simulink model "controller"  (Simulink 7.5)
settings: Solver=FixedStepDiscrete  StartTime=0.0  StopTime=Inf  FixedStep=0.002  RelTol=1e-3
PostLoadFcn:
  | , if any(exist('dsrtsu_mdlpostloadfcn', 'file') == [2, 3, 6]), try dsrtsu_mdlpostloadfcn('Execute', bdroot); catch fprintf('Error in PostLoadFcn (dsrtsu_mdlpostloadfcn) for model "%s":
  |  %s
  | ', bdroot, lasterr); end, end,
libraries: rtilib1103 x5, simulink x1

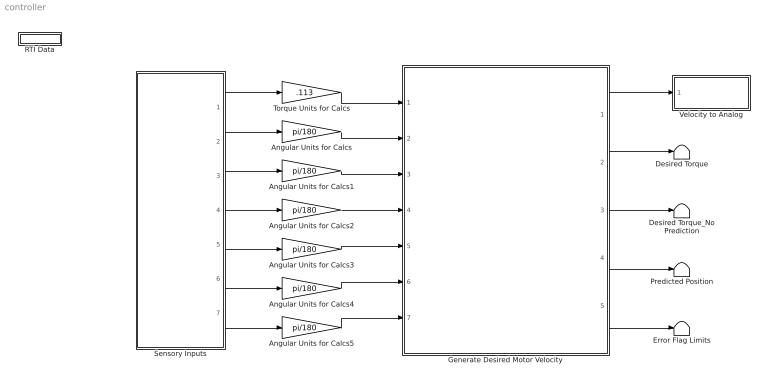
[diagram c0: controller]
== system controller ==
  Angular Units for Calcs{,1..5} (6 alike) : Gain  Gain=pi/180
  Desired Torque : Terminator
  Desired Torque_No Prediction : Terminator
  Error Flag Limits : Terminator
  Generate Desired Motor Velocity : Subsystem
  Predicted Position : Terminator
  RTI Data : Subsystem  Tag=struct('RTIDataServer',struct('RTIDataServerVs','2','RTIModelDescription','struct(''main'',''controller'',''sub'','''',''isMp'',0)'))  LoadFcn="if exist('rtidc'), try,  rtidc('DataHostBlockClbLoad', gcbh); catch, disp(['Warning: ''LoadFcn'' for RTI Data block failed: ' lasterr]); end, end,"
  Sensory Inputs : Subsystem
  Torque Units for Calcs : Gain  Gain=.113
  Velocity to Analog : Subsystem
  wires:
  Generate Desired Motor Velocity/1(Desired Velocity) -> Velocity to Analog/1(Velocity)
  Sensory Inputs/1(Ankle Torque) -> Torque Units for Calcs/1
  Sensory Inputs/2(Ankle Position) -> Angular Units for Calcs/1
  Sensory Inputs/3(Ankle Velocity) -> Angular Units for Calcs1/1
  Sensory Inputs/4(Sprocket Position) -> Angular Units for Calcs2/1
  Sensory Inputs/5(Sprocket Velocity) -> Angular Units for Calcs3/1
  Sensory Inputs/6(Motor Position) -> Angular Units for Calcs4/1
  Sensory Inputs/7(Motor Velocity) -> Angular Units for Calcs5/1
  Torque Units for Calcs/1 -> Generate Desired Motor Velocity/1(Ankle Torque)
  Angular Units for Calcs/1 -> Generate Desired Motor Velocity/2(Ankle Position)
  Angular Units for Calcs1/1 -> Generate Desired Motor Velocity/3(Ankle Velocity)
  Angular Units for Calcs2/1 -> Generate Desired Motor Velocity/4(Sprocket Position)
  Angular Units for Calcs3/1 -> Generate Desired Motor Velocity/5(Sprocket Velocity)
  Angular Units for Calcs4/1 -> Generate Desired Motor Velocity/6(Motor Position)
  Angular Units for Calcs5/1 -> Generate Desired Motor Velocity/7(Motor Velocity)
  Generate Desired Motor Velocity/2(Desired Torque) -> Desired Torque/1
  Generate Desired Motor Velocity/3(Desired Torque_No Prediction) -> Desired Torque_No Prediction/1
  Generate Desired Motor Velocity/4(Predicted Position) -> Predicted Position/1
  Generate Desired Motor Velocity/5(Error Flag_Limits) -> Error Flag Limits/1

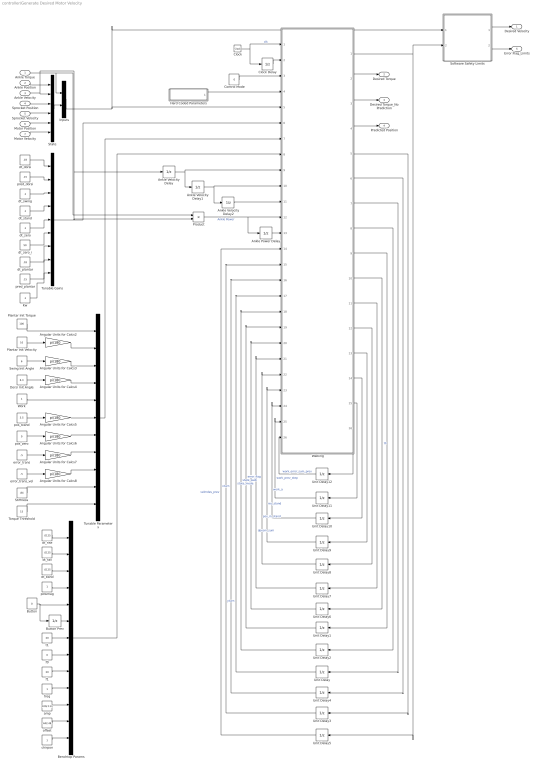
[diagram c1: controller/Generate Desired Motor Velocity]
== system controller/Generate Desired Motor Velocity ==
  Ankle Torque : Inport
  Ankle Position : Inport  Port=2
  Ankle Velocity : Inport  Port=3
  Sprocket Position : Inport  Port=4
  Sprocket Velocity : Inport  Port=5
  Motor Position : Inport  Port=6
  Motor Velocity : Inport  Port=7
  Angular Units for Calcs{2..8} (7 alike) : Gain  Gain=pi/180
  Ankle Power Delay : UnitDelay  SampleTime=0.002
  Ankle Velocity Delay : UnitDelay  SampleTime=0.002
  Ankle Velocity Delay1 : UnitDelay  SampleTime=0.002
  Ankle Velocity Delay2 : UnitDelay  SampleTime=0.002
  Benchtop Params : Mux  Inputs=13
  Button : Constant  Value=0
  Button Prev : UnitDelay  X0=1  SampleTime=0.002
  Clock : Clock
  Clock Delay : UnitDelay  SampleTime=0.002
  Control Mode : Constant  Value=0  SampleTime=.002
  Dorsi Init Angle : Constant  Value=6.3  SampleTime=.002
  Hard Coded Parameters : Stateflow chart  TreatAsAtomicUnit=on
  Inputs : Mux  Inputs=2
  Kw : Constant  Value=.1  SampleTime=.002
  Plantar Init Torque : Constant  Value=100  SampleTime=.002
  Plantar Init Velocity : Constant  Value=10  SampleTime=.002
  Product : Product  OutDataType=fixdt(1, 16)  OutScaling=2^0
  Software Safety Limits : Stateflow chart  TreatAsAtomicUnit=on
  State : Mux  Inputs=6
  Stiffness : Constant  Value=.84  SampleTime=.002
  Swing Init Angle : Constant  Value=6  SampleTime=.002
  Torque Threshold : Constant  Value=15  SampleTime=.002
  Tunable Gains : Mux  Inputs=9
  Tunable Parameters : Mux  Inputs=11
  Unit Delay{,1..12} (13 alike) : UnitDelay  SampleTime=0.002
  Walking : Stateflow chart  TreatAsAtomicUnit=on
  Work : Constant  SampleTime=.002
  amp : Constant  Value=100/.113  SampleTime=.002
  chirpon : Constant  SampleTime=.002
  dt_band : Constant  Value=.0125  SampleTime=.002
  dt_dorsi : Constant  Value=.03  SampleTime=.002
  dt_fall : Constant  Value=.0125  SampleTime=.002
  dt_plantar : Constant  Value=.03  SampleTime=.002
  dt_rise : Constant  Value=.0125  SampleTime=.002
  dt_stand : Constant  Value=.1  SampleTime=.002
  dt_swing : Constant  Value=.1  SampleTime=.002
  dt_zero : Constant  Value=.1  SampleTime=.002
  dt_zero_i : Constant  Value=50  SampleTime=.002
  error_trans : Constant  Value=.5  SampleTime=.002
  error_trans_vel : Constant  Value=.5  SampleTime=.002
  f0 : Constant  Value=0  SampleTime=.002
  f1 : Constant  Value=20  SampleTime=.002
  freq : Constant  SampleTime=.002
  offset : Constant  Value=442.48  SampleTime=.002
  pos_stand : Constant  Value=3.5  SampleTime=.002
  pos_zero : Constant  Value=0  SampleTime=.002
  powmag : Constant  SampleTime=.002
  pred_dorsi : Constant  Value=.15  SampleTime=.002
  pred_plantar : Constant  Value=.15  SampleTime=.002
  t1 : Constant  Value=20  SampleTime=.002
  Desired Velocity : Outport
  Desired Torque : Outport  Port=2
  Desired Torque_No Prediction : Outport  Port=3
  Predicted Position : Outport  Port=4
  Error Flag_Limits : Outport  Port=5
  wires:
  Walking/7(next_state_mode) -> Unit Delay/1
  Unit Delay/1 -> Walking/17(state_mode)  "state_mode"
  Walking/5(next_yturn) -> Unit Delay3/1
  Walking/6(next_xturn) -> Unit Delay4/1
  Unit Delay4/1 -> Walking/16(xturn)  "xturn"
  Ankle Velocity Delay/1 -> Ankle Velocity Delay1/1, Walking/9(vel_a_prev1)
  Ankle Velocity Delay1/1 -> Ankle Velocity Delay2/1, Walking/10(vel_a_prev2)
  Software Safety Limits/1(velmdes_lim) -> Desired Velocity/1
  Plantar Init Torque/1 -> Tunable Parameters/1
  Plantar Init Velocity/1 -> Angular Units for Calcs2/1
  Swing Init Angle/1 -> Angular Units for Calcs3/1
  Dorsi Init Angle/1 -> Angular Units for Calcs4/1
  dt_dorsi/1 -> Tunable Gains/1
  pred_dorsi/1 -> Tunable Gains/2
  Work/1 -> Tunable Parameters/5
  Hard Coded Parameters/1(p) -> Walking/4(params)
  Tunable Parameters/1 -> Walking/7(params_t)
  Tunable Gains/1 -> Walking/6(gains)
  pos_stand/1 -> Angular Units for Calcs5/1
  pos_zero/1 -> Angular Units for Calcs6/1
  dt_swing/1 -> Tunable Gains/3
  Ankle Position/1 -> State/1
  Ankle Velocity/1 -> State/2, Ankle Velocity Delay/1, Product/2
  Sprocket Position/1 -> State/3
  Sprocket Velocity/1 -> State/4
  Motor Position/1 -> State/5
  Motor Velocity/1 -> State/6
  Ankle Torque/1 -> Inputs/1, Product/1
  State/1 -> Inputs/2
  Inputs/1 -> Walking/5(inputs), Software Safety Limits/1(inputs)
  error_trans/1 -> Angular Units for Calcs7/1
  Angular Units for Calcs2/1 -> Tunable Parameters/2
  Angular Units for Calcs3/1 -> Tunable Parameters/3
  Angular Units for Calcs4/1 -> Tunable Parameters/4
  Angular Units for Calcs5/1 -> Tunable Parameters/6
  Angular Units for Calcs6/1 -> Tunable Parameters/7
  Angular Units for Calcs7/1 -> Tunable Parameters/8
  Unit Delay3/1 -> Walking/15(yturn)  "yturn"
  dt_stand/1 -> Tunable Gains/4
  dt_rise/1 -> Benchtop Params/1
  dt_fall/1 -> Benchtop Params/2
  dt_band/1 -> Benchtop Params/3
  powmag/1 -> Benchtop Params/4
  Button/1 -> Benchtop Params/5, Button Prev/1
  Button Prev/1 -> Benchtop Params/6
  t1/1 -> Benchtop Params/7
  f0/1 -> Benchtop Params/8
  f1/1 -> Benchtop Params/9
  freq/1 -> Benchtop Params/10
  amp/1 -> Benchtop Params/11
  offset/1 -> Benchtop Params/12
  chirpon/1 -> Benchtop Params/13
  Stiffness/1 -> Tunable Parameters/10
  error_trans_vel/1 -> Angular Units for Calcs8/1
  Angular Units for Calcs8/1 -> Tunable Parameters/9
  dt_zero/1 -> Tunable Gains/5
  Benchtop Params/1 -> Walking/8(params_b)
  Walking/1(velmdes) -> Software Safety Limits/2(velmdes), Unit Delay5/1
  Walking/2(taudes) -> Desired Torque/1
  Walking/3(taudes_nopred) -> Desired Torque_No Prediction/1
  Walking/4(pos_a_pred) -> Predicted Position/1
  Ankle Velocity Delay2/1 -> Walking/11(vel_a_prev3)
  Walking/8(next_state_walk) -> Unit Delay2/1
  Unit Delay2/1 -> Walking/18(state_walk)  "state_walk"
  Walking/9(next_error_flag) -> Unit Delay1/1
  Unit Delay1/1 -> Walking/19(error_flag)  "error_flag"
  Unit Delay5/1 -> Walking/14(velmdes_prev)  "velmdes_prev"
  Walking/10(t0) -> Unit Delay6/1  "t0"
  Unit Delay6/1 -> Walking/20(t0_prev)
  Software Safety Limits/2(error_flag_lim) -> Error Flag_Limits/1
  dt_zero_i/1 -> Tunable Gains/6
  Unit Delay7/1 -> Walking/21(dposm_sum)  "dposm_sum"
  Walking/11(dposm_sum_next) -> Unit Delay7/1
  Walking/12(pos_m_stand_next) -> Unit Delay8/1
  Unit Delay8/1 -> Walking/22(pos_m_stand)  "pos_m_stand"
  Unit Delay9/1 -> Walking/23(rec_stand)  "rec_stand"
  Walking/13(rec_stand_next) -> Unit Delay9/1
  Unit Delay10/1 -> Walking/24(work_a)  "work_a"
  Walking/14(next_work_a) -> Unit Delay10/1
  Control Mode/1 -> Walking/3(mode)
  Ankle Power Delay/1 -> Walking/13(pow_prev)
  Product/1 -> Ankle Power Delay/1, Walking/12(pow)  "Ankle Power"
  Clock/1 -> Walking/1(clk), Clock Delay/1  "clk"
  Clock Delay/1 -> Walking/2(clk_prev)
  dt_plantar/1 -> Tunable Gains/7
  pred_plantar/1 -> Tunable Gains/8
  Torque Threshold/1 -> Tunable Parameters/11
  Walking/15(work_step) -> Unit Delay11/1
  Unit Delay11/1 -> Walking/25(work_prev_step)  "work_prev_step"
  Kw/1 -> Tunable Gains/9
  Walking/16(work_error_sum) -> Unit Delay12/1
  Unit Delay12/1 -> Walking/26(work_error_sum_prev)  "work_error_sum_prev"

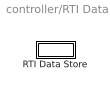
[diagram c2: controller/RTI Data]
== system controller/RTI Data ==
  RTI Data Store : Subsystem  Tag=struct('private',struct('version',struct('dsVer',uint32(2),'dsVerCreation',uint32(2),'RTI',struct('ver','6.6','type','RTI1103')),'access',struct('type','Model','isPerm',1,'created',['12-Aug-2011 17:25:08'],'modified',['25-Oct-2012 11:39:04'],'location','')),'public',struct('main',struct('data',[]),'sub',struct('name',{{'controller'}},'data',{{struct('TH',struct('thTaskInfo',struct('taskType',{'TIM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

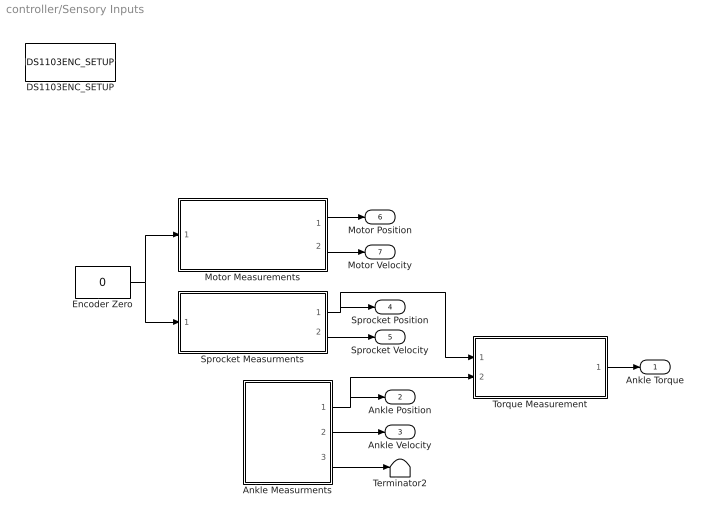
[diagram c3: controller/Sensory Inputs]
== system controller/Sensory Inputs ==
  Ankle Measurments : Subsystem
  DS1103ENC_SETUP : rtilib1103/DS1103 MASTER PPC/DS1103ENC_SETUP  SystemSampleTime=-1  EncRange=0  Reserved1=[]  Reserved2=[]  Reserved3=[]  Reserved4=[]  DialogFcn=gui1103enc_setup  UnitName={ 'DS1103ENC_SETUP' }  UnitValues={ [] }  DSProperties=struct('RTI',struct('Version',uint32(1),'BlockType',struct('isSLSource',uint8(0),'isSLSink',uint8(0),'isHWSource',uint8(0),'isHWSink',uint8(0),'isSetup',uint8(0),'isInline',uint8(1),'isNonInline',uint8(0),'isInterrupt',uint8(0),'isChannelwise',uint8(0)),'IOBoardType','DS1103MASTER','UnitType','ENC','Identifier','ENCMASTER','DialogType','ML','BlockSet','NONE','SlaveProcessor','NONE'))
  Encoder Zero : Constant  Value=0
  Motor Measurements : Subsystem
  Sprocket Measurments : Subsystem
  Terminator2 : Terminator
  Torque Measurement : Stateflow chart  TreatAsAtomicUnit=on
  Ankle Torque : Outport
  Ankle Position : Outport  Port=2
  Ankle Velocity : Outport  Port=3
  Sprocket Position : Outport  Port=4
  Sprocket Velocity : Outport  Port=5
  Motor Position : Outport  Port=6
  Motor Velocity : Outport  Port=7
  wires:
  Torque Measurement/1(tau) -> Ankle Torque/1
  Ankle Measurments/1(Ankle Position) -> Ankle Position/1, Torque Measurement/2(pos)
  Ankle Measurments/2(Ankle Velocity) -> Ankle Velocity/1
  Sprocket Measurments/1(Sprocket Position) -> Sprocket Position/1, Torque Measurement/1(pos_s)
  Sprocket Measurments/2(Sprocket Velocity) -> Sprocket Velocity/1
  Motor Measurements/2(Motor Velocity) -> Motor Velocity/1
  Ankle Measurments/3(Encoder Voltage) -> Terminator2/1
  Motor Measurements/1(Motor Position) -> Motor Position/1
  Encoder Zero/1 -> Motor Measurements/1(Button), Sprocket Measurments/1(Button)

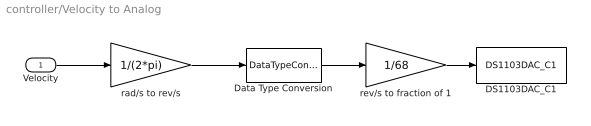
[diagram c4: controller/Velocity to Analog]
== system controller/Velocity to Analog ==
  Velocity : Inport
  DS1103DAC_C1 : rtilib1103/DS1103 MASTER PPC/DS1103DAC_C1  SystemSampleTime=-1  ChannelNo=1  InitValue=0  TermMode=1  TermValue=0  Reserved1=[]  Reserved2=[]  Reserved3=[]  Reserved4=[]  DialogFcn=gui1103dac  UnitName={ 'DS1103DAC_C' }  UnitValues={ 1 }  DSProperties=struct('RTI',struct('Version',uint32(1),'BlockType',struct('isSLSource',uint8(0),'isSLSink',uint8(1),'isHWSource',uint8(0),'isHWSink',uint8(1),'isSetup',uint8(0),'isInline',uint8(1),'isNonInline',uint8(0),'isInterrupt',uint8(0),'isChannelwise',uint8(1)),'IOBoardType','DS1103MASTER','UnitType','DAC','Identifier','DAC','DialogType','ML','BlockSet','NONE','SlaveProcessor','NONE'))
  Data Type Conversion : DataTypeConversion  OutDataTypeMode=double  OutDataTypeStr=double
  rad/s to rev/s : Gain  Gain=1/(2*pi)
  rev/s to fraction of 1 : Gain  Gain=1/68
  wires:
  Data Type Conversion/1 -> rev/s to fraction of 1/1
  rev/s to fraction of 1/1 -> DS1103DAC_C1/1
  Velocity/1 -> rad/s to rev/s/1
  rad/s to rev/s/1 -> Data Type Conversion/1

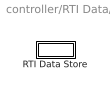
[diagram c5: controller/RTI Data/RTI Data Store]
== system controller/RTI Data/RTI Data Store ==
  RTI Data Store : Subsystem

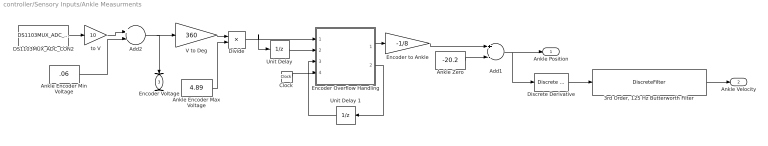
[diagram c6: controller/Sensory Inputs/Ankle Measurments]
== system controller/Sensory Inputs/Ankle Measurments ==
  "3rd Order, 125 Hz Butterworth Filter" : DiscreteFilter  Numerator=[0.1667 0.5000 0.5000 0.1667]  Denominator=[1.0000 -0.0000 0.3333 -0.0000]
  Add1 : Sum  Inputs=+-
  Add2 : Sum  Inputs=+-
  Ankle Encoder Max Voltage : Constant  Value=4.89
  Ankle Encoder Min Voltage : Constant  Value=.06
  Ankle Zero : Constant  Value=-20.2
  Clock : Clock
  DS1103MUX_ADC_CON2 : rtilib1103/DS1103 MASTER PPC/DS1103MUX_ADC_CON1  SystemSampleTime=-1  ConverterNo=2  ChannelNos=1  TimerAPreTrigger=0  Reserved2=[]  Reserved3=[]  Reserved4=[]  DialogFcn=gui1103mux_adc  UnitName={ 'DS1103MUX_ADC_CON' }  UnitValues={ 2 }  DSProperties=struct('RTI',struct('Version',uint32(1),'BlockType',struct('isSLSource',uint8(1),'isSLSink',uint8(0),'isHWSource',uint8(1),'isHWSink',uint8(0),'isSetup',uint8(0),'isInline',uint8(1),'isNonInline',uint8(0),'isInterrupt',uint8(0),'isChannelwise',uint8(0)),'IOBoardType','DS1103MASTER','UnitType','ADC','Identifier','ADCMUX','DialogType','ML','BlockSet','NONE','SlaveProcessor','NONE'))
  Discrete Derivative : simulink/Discrete/Discrete Derivative  SystemSampleTime=-1  gainval=1.0  ICPrevScaledInput=0.0  OutMin=[]  OutMax=[]  OutDataType=fixdt(1, 16)  OutScaling=2^-10  DoSatur=off
  Divide : Product  Inputs=*/
  Encoder Overflow Handling : Stateflow chart  TreatAsAtomicUnit=on
  Encoder to Ankle : Gain  Gain=-1/8
  Unit Delay : UnitDelay  SampleTime=.002
  Unit Delay 1 : UnitDelay  SampleTime=.002
  V to Deg : Gain  Gain=360
  to V : Gain  Gain=10
  Ankle Position : Outport
  Ankle Velocity : Outport  Port=2
  Encoder Voltage : Outport  Port=3
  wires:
  Discrete Derivative/1 -> "3rd Order, 125 Hz Butterworth Filter"/1
  Encoder to Ankle/1 -> Add1/1
  Ankle Zero/1 -> Add1/2
  Encoder Overflow Handling/2(rev) -> Unit Delay 1/1
  Unit Delay 1/1 -> Encoder Overflow Handling/3(rev_prev)
  DS1103MUX_ADC_CON2/1 -> to V/1
  Unit Delay/1 -> Encoder Overflow Handling/2(in_prev)
  Encoder Overflow Handling/1(out) -> Encoder to Ankle/1
  Clock/1 -> Encoder Overflow Handling/4(clk)
  Add1/1 -> Ankle Position/1, Discrete Derivative/1
  to V/1 -> Add2/1
  Add2/1 -> V to Deg/1, Encoder Voltage/1
  V to Deg/1 -> Divide/1
  Ankle Encoder Max Voltage/1 -> Divide/2
  Divide/1 -> Encoder Overflow Handling/1(in), Unit Delay/1
  Ankle Encoder Min Voltage/1 -> Add2/2
  "3rd Order, 125 Hz Butterworth Filter"/1 -> Ankle Velocity/1

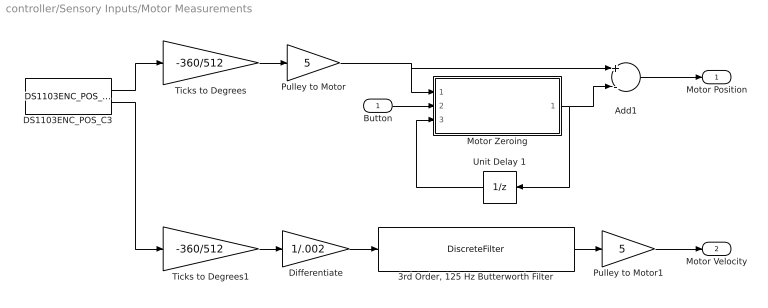
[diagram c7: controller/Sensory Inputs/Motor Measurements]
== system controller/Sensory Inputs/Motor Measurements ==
  Button : Inport  OutDataType=fixdt(1, 16)  OutScaling=2^0
  "3rd Order, 125 Hz Butterworth Filter" : DiscreteFilter  Numerator=[0.1667 0.5000 0.5000 0.1667]  Denominator=[1.0000 -0.0000 0.3333 -0.0000]
  Add1 : Sum  Inputs=+-
  DS1103ENC_POS_C3 : rtilib1103/DS1103 MASTER PPC/DS1103ENC_POS_C1  SystemSampleTime=-1  ChannelNo=3  PosValue=0  Reserved1=[]  Reserved2=[]  Reserved3=[]  Reserved4=[]  DialogFcn=gui1103enc_pos  UnitName={ 'DS1103ENC_POS_C' }  UnitValues={ 3 }  DSProperties=struct('RTI',struct('Version',uint32(1),'BlockType',struct('isSLSource',uint8(1),'isSLSink',uint8(0),'isHWSource',uint8(1),'isHWSink',uint8(0),'isSetup',uint8(0),'isInline',uint8(1),'isNonInline',uint8(0),'isInterrupt',uint8(0),'isChannelwise',uint8(1)),'IOBoardType','DS1103MASTER','UnitType','ENC','Identifier','ENCPOSCH','DialogType','ML','BlockSet','NONE','SlaveProcessor','NONE'))
  Differentiate : Gain  Gain=1/.002
  Motor Zeroing : Stateflow chart  TreatAsAtomicUnit=on
  Pulley to Motor : Gain  Gain=5
  Pulley to Motor1 : Gain  Gain=5
  Ticks to Degrees : Gain  Gain=-360/512
  Ticks to Degrees1 : Gain  Gain=-360/512
  Unit Delay 1 : UnitDelay  SampleTime=.002
  Motor Position : Outport
  Motor Velocity : Outport  Port=2
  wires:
  DS1103ENC_POS_C3/1 -> Ticks to Degrees/1
  DS1103ENC_POS_C3/2 -> Ticks to Degrees1/1
  Ticks to Degrees1/1 -> Differentiate/1
  Differentiate/1 -> "3rd Order, 125 Hz Butterworth Filter"/1
  Pulley to Motor1/1 -> Motor Velocity/1
  "3rd Order, 125 Hz Butterworth Filter"/1 -> Pulley to Motor1/1
  Add1/1 -> Motor Position/1
  Ticks to Degrees/1 -> Pulley to Motor/1
  Motor Zeroing/1(mpz) -> Unit Delay 1/1, Add1/2
  Button/1 -> Motor Zeroing/2(button)
  Unit Delay 1/1 -> Motor Zeroing/3(mpz_prev)
  Pulley to Motor/1 -> Add1/1, Motor Zeroing/1(pos_m)

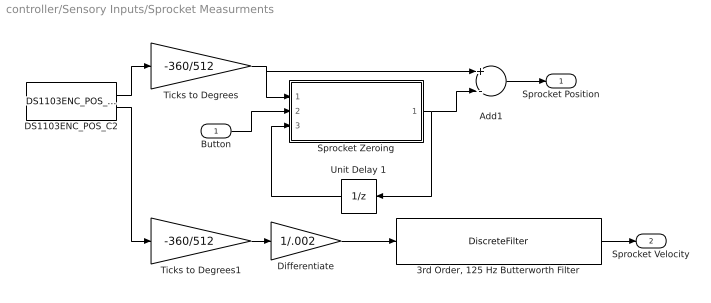
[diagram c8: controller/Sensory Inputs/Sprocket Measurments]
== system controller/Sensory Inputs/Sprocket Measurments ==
  Button : Inport  OutDataType=fixdt(1, 16)  OutScaling=2^0
  "3rd Order, 125 Hz Butterworth Filter" : DiscreteFilter  Numerator=[0.1667 0.5000 0.5000 0.1667]  Denominator=[1.0000 -0.0000 0.3333 -0.0000]
  Add1 : Sum  Inputs=+-
  DS1103ENC_POS_C2 : rtilib1103/DS1103 MASTER PPC/DS1103ENC_POS_C1  SystemSampleTime=-1  ChannelNo=2  PosValue=0  Reserved1=[]  Reserved2=[]  Reserved3=[]  Reserved4=[]  DialogFcn=gui1103enc_pos  UnitName={ 'DS1103ENC_POS_C' }  UnitValues={2}  DSProperties=struct('RTI',struct('Version',uint32(1),'BlockType',struct('isSLSource',uint8(1),'isSLSink',uint8(0),'isHWSource',uint8(1),'isHWSink',uint8(0),'isSetup',uint8(0),'isInline',uint8(1),'isNonInline',uint8(0),'isInterrupt',uint8(0),'isChannelwise',uint8(1)),'IOBoardType','DS1103MASTER','UnitType','ENC','Identifier','ENCPOSCH','DialogType','ML','BlockSet','NONE','SlaveProcessor','NONE'))
  Differentiate : Gain  Gain=1/.002
  Sprocket Zeroing : Stateflow chart  TreatAsAtomicUnit=on
  Ticks to Degrees : Gain  Gain=-360/512
  Ticks to Degrees1 : Gain  Gain=-360/512
  Unit Delay 1 : UnitDelay  SampleTime=.002
  Sprocket Position : Outport
  Sprocket Velocity : Outport  Port=2
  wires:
  Add1/1 -> Sprocket Position/1
  Ticks to Degrees/1 -> Add1/1, Sprocket Zeroing/1(pos_s)
  Differentiate/1 -> "3rd Order, 125 Hz Butterworth Filter"/1
  Ticks to Degrees1/1 -> Differentiate/1
  DS1103ENC_POS_C2/2 -> Ticks to Degrees1/1
  DS1103ENC_POS_C2/1 -> Ticks to Degrees/1
  "3rd Order, 125 Hz Butterworth Filter"/1 -> Sprocket Velocity/1
  Sprocket Zeroing/1(spz) -> Unit Delay 1/1, Add1/2
  Button/1 -> Sprocket Zeroing/2(button)
  Unit Delay 1/1 -> Sprocket Zeroing/3(spz_prev)

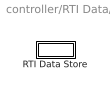
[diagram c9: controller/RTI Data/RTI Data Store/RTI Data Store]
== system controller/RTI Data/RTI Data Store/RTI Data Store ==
  RTI Data Store : Subsystem

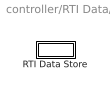
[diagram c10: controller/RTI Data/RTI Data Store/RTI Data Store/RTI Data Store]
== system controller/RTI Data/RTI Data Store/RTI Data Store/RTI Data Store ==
  RTI Data Store : Subsystem

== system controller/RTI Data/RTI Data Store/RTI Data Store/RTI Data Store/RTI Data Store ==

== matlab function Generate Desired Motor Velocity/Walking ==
function [velmdes,taudes,taudes_nopred,pos_a_pred,...
          next_yturn,next_xturn,next_state_mode,next_state_walk,next_error_flag,t0,dposm_sum_next,pos_m_stand_next,rec_stand_next,next_work_a,work_step,work_error_sum] = ...
    fcn(clk,clk_prev,mode,params,inputs,gains,params_t,params_b,...
        vel_a_prev1,vel_a_prev2,vel_a_prev3,pow,pow_prev,...
        velmdes_prev,yturn,xturn,state_mode,state_walk,error_flag,t0_prev,dposm_sum,pos_m_stand,rec_stand,work_a,work_prev_step,work_error_sum_prev)

%% ------------------
%% UPACK MUXED INPUTS
%% ------------------

% hard coded parameters
[Rg] = params(1);
[RgRf] = params(2);
[Ks] = params(3);
[Ka] = params(4);
[Ktr] = params(5);

% sensory measurments
[tau] = inputs(1);
[pos_a] = inputs(2);
[vel_a] = inputs(3);
[pos_s] = inputs(4);
[vel_s] = inputs(5);
[pos_m] = inputs(6);
[vel_m] = inputs(7);

% tunable control gains
[dt_dorsi] = gains(1);
[pred_dorsi] = gains(2);
[dt_swing] = gains(3);
[dt_stand] = gains(4);
[dt_zero] = gains(5);
[dt_zero_i] = gains(6);
[dt_plantar] = gains(7);
[pred_plantar] = gains(8);
[Kw] = gains(9);

% tunable parameters
[plantar_trans_tor] = params_t(1);
[plantar_trans_vel] = params_t(2);
[swing_trans] = params_t(3);
[dorsi_trans] = params_t(4);
[W] = params_t(5);
[pos_stand] = params_t(6);
[pos_zero] = params_t(7);
[error_trans] = params_t(8);
[error_trans_vel] = params_t(9);
[K] = params_t(10);
[tau_thresh] = params_t(11);

% tunable parameters for benchtop testing
[dt_rise] = params_b(1);
[dt_fall] = params_b(2);
[dt_band] = params_b(3);
[powmag] = params_b(4);
[button] = params_b(5);
[button_prev] = params_b(6);
[t1] = params_b(7);
[f0] = params_b(8);
[f1] = params_b(9);
[freq] = params_b(10);
[amp] = params_b(11);
[offset] = params_b(12);
[chirpon] = params_b(13);

%% ----------
%% END UNPACK
%% ----------

%% ------------------
%% MODE STATE MACHINE
%% ------------------

ZERO = 0; STAND = 1; WALK = 2; POWER = 3; STEP = 4; BAND = 5; CAL = 10; % State names
enable_walk = 0; % Default to turn off walkinig state machine
t0 = t0_prev; dposm_sum_next = dposm_sum; pos_m_stand_next = pos_m_stand; rec_stand_next = rec_stand; % Default propogations

switch state_mode
    case ZERO % servo ankle position to zero
        %% Output
        dposa = pos_zero - pos_a; % difference between anke position and zero
        dposm = dposa * RgRf; % multiply by gain to get ~motor position
        % Motor command
        if (abs(dposa) > error_trans) % if error is larger than some tolerance
            velmdes = dposm / dt_zero / 3; % weak p control if far away
            dposm_sum_next = 0; % don't integrate position error
        else
            dposm_sum_next = dposm_sum + dposm; % integrate position error
            velmdes = dposm / dt_zero + dposm_sum / dt_zero_i; % stronger p + i control if close to zero
        end
        %% Transition
        next_state_mode = mode; % switch modes immediately if commanded to
        rec_stand_next = 0; % for transition to standing mode
    case STAND % servo motor position to the standing position
        %% Output
        if (abs(pos_stand-pos_a) > error_trans) && rec_stand == 0 % weak p control of ankle angle if far away from goal
            dposa = pos_stand - pos_a; % difference between ankle position and desired no-load ankle position during standing
            dposm = dposa * RgRf; % multiply by gain to get ~motor position
            velmdes = dposm / dt_zero / 3; % weak p control
        else
            if(rec_stand == 0) % if we're transitioning to standing mode and we're not at the goal
                rec_stand_next = 1; % record new goal           
                pos_m_stand_next = pos_m; % record motor position that correlates with desired ankle position
            end
            dposm = pos_m_stand - pos_m; % difference between motor position and recorded goal
            velmdes = dposm / dt_stand; % p control of motor position
        end
        %% Transition
        next_state_mode = mode; % switch modes immediately if commanded to
    case WALK % enable walking state machine to control motor command
        %% Output
        if mode == WALK
            enable_walk = 1; % Enable walking controller
        else
            enable_walk = 0; % Default to turn off walkinig state machine
        end
        velmdes = 0; % need to command something for this clock cycle
        %% Transition
        next_state_mode = mode; % switch modes immediately if commanded to
    case POWER % open-loop peak power (scary)
        %% Output
        velmmax = powmag*65*2*pi; % move at maximum velocity, scaled by powmag
        velmdes = velmmax; 
        %% Transition
        next_state_mode = mode; % switch modes immediately if commanded to
        rec_stand_next = 0;
    case STEP % torque-control step response
        %% Output
        mag = 100;
        step = button*mag; % step response at the command of button with maginute of mag
        if button > 0; % allow for different gains to be used for upward and downward steps
            dt = dt_rise;
        else
            dt = dt_fall;
        end
        if step == 0 % command some small torque when the button is released, to avoid drift
            step = 200*.113;
        end
        dtau = step - tau; % compute torque error
        dpos_s = dtau / Ks; % calculate desired change in sprocket position given torque error
        dpos_m = Rg * dpos_s + dtau/Ktr; % calculate desired motor position
        % Motor command
        velmdes = dpos_m / dt; % compute commanded motor velocity
        % Control reference
        taudes = step; % just for post-hoc plotting
        %% Transition
        next_state_mode = mode; % switch modes immediately if commanded to
        rec_stand_next = 0;
    case BAND % torque-control chirp response
        %% Output
        if chirpon == 0;
            bwtau = (amp-offset)*(sin(clk*freq*2*pi)+1)/2 + offset; % if desired, command sinusoid of constant frequency
        else
            if button == 1 % otherwise, command a chirp
                if button_prev == 0 % set time to zero at time of button press
                    t0 = clk;
                end
                clk = max(clk-t0,0);
                if clk >= t1; % stop the chirp if we exceed t1
                    over = 0;
                else
                    over = 1;
                end
                f = f0 + (f1-f0)/t1*clk; % compute linearly increasing chirp frequency
                bwtau = over*(amp-offset)*(-cos(clk*f/2*2*pi)+1)/2 + offset; % compute chirp torque
            else
                bwtau = offset; % command constant torque about which chirp oscillates if button released
            end
        end

        dtau = bwtau - tau; % compute torque error
        dpos_s = dtau / Ks; % calculate desired change in sprocket position given torque error
        dpos_m = Rg * dpos_s + dtau/Ktr; % calculate desired motor position
        % Motor command
        velmdes = dpos_m / dt_band; % compute commanded motor velocity
        % Control reference
        taudes = bwtau; % just for post-hoc plotting
        %% Transition
        next_state_mode = mode; % switch modes immediately if commanded to
        rec_stand_next = 0;
    case CAL % auto calibration
        %% Output
        % Motor command
        if pos_a < -15*pi/180 % if negetive angle limit is reached, move in positive direction
            velmdes = 1;
        elseif pos_s > 175*pi/180 % if positive sprocket limit is reached, move in negative direction
            velmdes = -1;
        else
            velmdes = velmdes_prev; % keep doing what we were doing if not at limit
        end
        %% Transition
        next_state_mode = mode; % switch modes immediately if commanded to
        rec_stand_next = 0;
    otherwise
        velmdes = 0; rec_stand_next = 0;
        next_state_mode = state_mode;
end

%% -----------
%% END MODE SM
%% -----------

%% ------------------
%% WALK STATE MACHINE
%% ------------------

WAIT = 0; DORSI = 1; PLANTAR = 2; SWING = 3; % State names
CLEAR = 0; EARLYPLANT = 1; SLOWSWING = 2; % Error flags

next_yturn = yturn; next_xturn = xturn; next_error_flag = error_flag; next_state_walk = state_walk; work_error_sum = work_error_sum_prev; % Default propogation
taudes = 0; taudes_nopred = 0; pos_a_pred = 0; work_step = 0; % Some defaults

switch state_walk
    case WAIT % do nothing
        % Output
        next_work_a = 0;
        % Transition
        if enable_walk == 1 % if state machine is not enabled, stay in wait, doing nothing
            next_state_walk = DORSI;
        else
            next_state_walk = WAIT;
        end
    case DORSI % track the dorsiflexion torque-angle relationship
        % Output (vm = kp1*tor_ankle_error+kp2*pos_ankle_error)
        if tau < tau_thresh % if we are below some torque threshold, position control motor, ala standing
            dposm = pos_m_stand - pos_m; % compute motor position error
            velmdes = dposm / dt_stand; % p control of motor position
            taudes = 0; % for post-hoc plotting
            next_work_a = 0; % don't start integrating work until tau exceeds and stays above tau_thresh
        else
            next_work_a = work_a + (pow+pow_prev)/2*(clk-clk_prev); % integrate ankle work
            [velmdes, taudes, pos_a_pred] = dorsi_vel(tau, pos_a, vel_a, dt_dorsi, Ks, Ka, Rg, Ktr, pred_dorsi, K); % compute reference torque for torque controller
            [temp,taudes_nopred,temp1] = dorsi_vel(tau, pos_a, vel_a, dt_dorsi, Ks, Ka, Rg, Ktr, 0, K); % compute reference torque without prediction
        end
        
        next_error_flag = CLEAR;
        
        % Transition
        if enable_walk == 1 % only take action if walking state machine is enabled
            if (tau > plantar_trans_tor) && ... % if we're in the second torque bump ...
               (vel_a > plantar_trans_vel) && (vel_a_prev1 > plantar_trans_vel) && ... % and velocity is increasing
               (vel_a_prev2 > plantar_trans_vel) && (vel_a_prev3 > plantar_trans_vel)
                next_state_walk = PLANTAR; % transition to plantarflexion
                next_yturn = taudes_nopred; % max torque/min angle of work loop set to point of transition to plantarflexion
                next_xturn = pos_a;
            end
        else
            next_state_walk = WAIT;
        end
    case PLANTAR % track the plantarflexion torque-angle relationship
        % Output (vm = kp1*tor_ankle_error+kp2*pos_ankle_error)
        if tau < tau_thresh % if we are below some torque threshold, stance is ending
            taudes = 0; % just for post-hoc plotting
            work_step = work_a; % record work supplied on this step
%             work_error_sum = (W - work_prev_step) + work_error_sum_prev; % integrate error between desired work and actual work on the previous step (currently not used)
            next_work_a = 0; % stop integrating work
        else
%             Cw = f(W) + Kw*work_error_sum; % Cw is some function of desired work + integral control to account for error in mapping / systematic torque control errors (currently not used)
            next_work_a = work_a + (pow+pow_prev)/2*(clk-clk_prev); % integrate work
            [velmdes, taudes, pos_a_pred] = plantar_vel(tau, pos_a, vel_a, dt_plantar, W, yturn, xturn, Ks, Ka, Rg, Ktr, pred_plantar, K); % compute reference torque for torque controller
            [temp,taudes_nopred,temp1] = plantar_vel(tau, pos_a, vel_a, dt_plantar, W, yturn, xturn, Ks, Ka, Rg, Ktr, 0, K); % compute reference torque without prediction
        end
        
        % Transition
        if enable_walk == 1 % only take action if walking state machine is enabled
            if taudes == 0; % if the toe is off the ground, go to swing
                next_state_walk = SWING;
            elseif (pos_a <= xturn) % if we switched to plantarflexion too early (due to an early positive bump in velocity) avoid problems by going back into dorsiflexion 
                next_error_flag = EARLYPLANT;
                next_state_walk = DORSI;
            end 
        else
            next_state_walk = WAIT;
        end
    case SWING % position servo the ankle to neutral configuration
        % Output (vm = kp*pos_ankle_error
        dposa = dorsi_trans - pos_a; % desired change in ankle position
        dposm = dposa * RgRf; % desired change in motor position
        velmdes = dposm / dt_swing; % position control ankle
        
        next_work_a = 0; % don't integrate work during swing
        
        % Transition
        if enable_walk == 1 % only take action if walking state machine is enabled
            if abs(pos_a-dorsi_trans) < error_trans % if the ankle is at the desired pre-touchdown position
                pos_m_stand_next = pos_m; % record motor position that correlates with this ankle position (will cause the motor to hold this position)
                next_state_walk = DORSI; % transition to dorsiflexion
            elseif tau > tau_thresh % if large torques appear during swing
                next_error_flag = SLOWSWING; % give warning that this is happening
                next_state_walk = DORSI; % and transition to dorsiflexion
            end
        else
            next_state_walk = WAIT;
        end
    otherwise
        velmdes = 0; next_work_a = 0;
        next_state_walk = WAIT;  
end

%% -----------
%% END WALK SM
%% -----------

return % end of fcn

% |-----------------------------------------|
% | Stance-Phase Motor Velocity Calculation |
% |-----------------------------------------|

function [velmdes, taudes, pos_a_dt] = dorsi_vel(tau, pos_a, vel_a, dt, Ks, Ka, Rg, Ktr, pred, K)
    % estimate of ankle state at future time
    dpos_a = vel_a*dt*pred;
    pos_a_dt = pos_a + dpos_a;
    
    % desired ankle torque at time control decisions will take effect     
    taudes = dorsi_torque_curve(pos_a_dt, K);
    
    % desired change in torque
    dtau = taudes - tau;
    
    % desired motor position, implied by desired future torque and ankle position 
    dpos_s = (dtau - Ka*dpos_a) / Ks; % change in sproket position
    dpos_m = Rg * dpos_s + dtau/Ktr; % change in motor position
    
    % this implies a desired velocity
    velmdes = dpos_m / dt;
return

function [velmdes, taudes, pos_a_dt] = plantar_vel(tau, pos_a, vel_a, dt, W, yturn, xturn, Ks, Ka, Rg, Ktr, pred, K)
    % estimate of ankle state at future time
    dpos_a = vel_a*dt*pred;
    pos_a_dt = pos_a + dpos_a;
    
    % desired ankle torque at time control decisions will take effect     
    taudes = plantar_torque_curve(pos_a_dt, W, yturn, xturn, K);
    
    % desired change in torque
    dtau = taudes - tau;
    
    % desired motor position, implied by desired future torque and ankle position 
    dpos_s = (dtau - Ka*dpos_a) / Ks; % change in sproket position
    dpos_m = Rg * dpos_s + dtau/Ktr; % change in motor position
    
    % this implies a desired velocity
    velmdes = dpos_m / dt;
return

% |---------------------------------------------------|
% | Ankle Position & Velocity vs. Torque Relationship |
% |----------------------------------------------------------------|
% | NOTE: See torquecurve.m for offline torque curve design sandbox| 
% |----------------------------------------------------------------|

function taudes = dorsi_torque_curve(pos_a, K)
    % hard-coded nodes on dorsiflexion curve
    xint1 = 0.11;   x1 = -0.10;    y1 = 65*K;
    yturn = 160*K;  xturn = -0.175;
    xint = xint1;   xadjust = x1;  yadjust = y1;
    
    % depending where we are on the curve, create a line in angle-torque space to follow
    if pos_a > xadjust      % if we're in the shallow part
        m = (0-yadjust)/(xint-xadjust);
        b = yadjust - xadjust*m;
    else                    % we're in the steeper part
        m = (yturn-yadjust)/(xturn-xadjust);
        b = yturn - xturn*m;
    end
    % desired torque is a linear fit on these terms
    taudes = [pos_a 1]*[m b]';
    
    % Disallow negative torques
    taudes = max(taudes,0);
return

function taudes = plantar_torque_curve(pos_a, Cw, yturn, xturn, K)
    % hard-coded nodes on dorsiflexion curve
    xint1 = 0.11;   x1 = -0.10;    y1 = 65*K;

    % Cw dependent nodes on plantarflexion curve
    if Cw >= 0 && Cw <= 1
        xint = xint1 + (0.22 - xint1)*Cw;
        xadjust = x1 + (0.03 - x1)*Cw;
        yadjust = y1 + (42*K - y1)*Cw;
    elseif Cw > 1 % for big positive work
        xint = .22; % fixed max plantar
        m = (.22-.03)/4; b = .03 - m; % denominator in m equation + 1 => Cw which gives max work
        xadjust = m*Cw + b;
        m = (yturn - 42*K)/4; b = 42*K - m;
        yadjust = m*Cw + b;
    else % for big negative work
        xint = .11; % fixed max plantar
        m = (xturn + .1)/-1.5; b = -.1; % denominator in m equation => Cw which gives min work
        xadjust = m*Cw + b;
        m = (-65*K)/-1.5; b = 65*K;
        yadjust = m*Cw + b;
    end
    
    % depending where we are on the curve, create a line in angle-torque space to follow
    if pos_a > xadjust      % if we're in the shallow part
        m = (0-yadjust)/(xint-xadjust);
        b = yadjust - xadjust*m;
    else                    % we're in the steeper part
        m = (yturn-yadjust)/(xturn-xadjust);
        b = yturn - xturn*m;
    end
    % desired torque is a linear fit on these terms
    taudes = [pos_a 1]*[m b]';
    
    % Disallow negative torques
    taudes = max(taudes,0);
return

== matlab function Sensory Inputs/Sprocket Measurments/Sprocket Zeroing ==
function spz = torqueseafun(pos_s,button,spz_prev)

if button
    spz = pos_s;
else
    spz = spz_prev;
end

return

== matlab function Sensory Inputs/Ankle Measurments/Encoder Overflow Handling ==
function [out,rev] = fcn(in,in_prev,rev_prev,clk)

if abs(in-in_prev) > 180 % if there is a big jump in encoder position (overflow)
    rev = rev_prev - sign(in-in_prev); % increment rev by +1 for 360 to 0 transition, -1 for 0 to 360
else
    rev = rev_prev;
end

out = in + 360 * rev; % add keep track of full revolutions of encoder and add to output

if(clk < .1)
    rev = 0;
end

return

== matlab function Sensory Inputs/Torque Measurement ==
function tau = torqueseafun(pos_s,pos)
%% ALL UNITS IN IN-LB & DEG
%% Refer to Dropbox/Prosthesis Testbed/Data Analysis/Stiffness Characterization

% ankle neutral angle setting constants
% Cap = [2.73306479968545e-07;-8.20921705057627e-06;0.121205272745540];
% Cap = [2.99453527654627e-07;-3.62907530653776e-05;0.123506206458447];
Cap = [.1246];%[.1271];
% Can = [6.41463967735540e-05;0.134691640977947];
% Can = [-4.27217678207691e-05;0.112822532443484];
Can = [.1203];%[.1191];

% calculate ankle neutral angle
if pos_s >= 0
%     ankle0 = [pos_s^3 pos_s^2 pos_s]*Cap;
    ankle0 = pos_s*Cap;
else
%     ankle0 = [pos_s^2 pos_s]*Can;
    ankle0 = pos_s*Can;
end

% ankle deflection is relative to neutral angle
ankledef = pos - ankle0;
% stiffness constant
% Ka = -89.6; % in-lb / deg
% Ka = -124.3036; % in-lb / deg
% Ka = -122.7278; % in-lb / deg
Ka = -115.59; % in-lb / deg

% torque is (approximated as) deflection times stiffness
tau = Ka*ankledef;

return

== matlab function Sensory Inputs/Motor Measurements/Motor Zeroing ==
function mpz = torqueseafun(pos_m,button,mpz_prev)

if button
    mpz = pos_m;
else
    mpz = mpz_prev;
end

return

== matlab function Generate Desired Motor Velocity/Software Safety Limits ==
function [velmdes_lim,error_flag_lim] = fcn(inputs,velmdes)

%% -----
%% UPACK
%% -----

% sensory measurments
[tau] = inputs(1);
[pos_a] = inputs(2);
[vel_a] = inputs(3);
[pos_s] = inputs(4);
[vel_s] = inputs(5);
[pos_m] = inputs(6);
[vel_m] = inputs(7);

%% ---------
%% END UNPACK
%% ---------

MAX_VEL = 1; MAX_TAU = 2; MAX_SPROCKET = 3; MAX_MOTOR = 4; % error flag definitions

% Software Limits Parameters 
tau_max = 1600*0.113;   % maximum allowable ankle torque, in Newton meters
pos_s_max = 195*pi/180; % 150 maximum allowable dorsiflexion angle (sprocket), in radians
velmax = 65*2*pi; % maximum allowable motor velocity, in radians per second

velmdes_lim = velmdes; % Default, do nothing
error_flag_lim = 0; % Default, no limits reached

% Limit maximum command velocity (saturate)
if velmdes > velmax
    velmdes_lim = velmax;
    error_flag_lim = MAX_VEL;
elseif velmdes < -velmax
    velmdes_lim = -velmax;
    error_flag_lim = MAX_VEL;
end

% Limit maximum measured torque
if tau > tau_max
    velmdes_lim = -1;
    error_flag_lim = MAX_TAU;
end

% Limit maximum sprocket plantarflexion angle
if pos_s > pos_s_max % If this then foot is likely off ground and in wrong state
    velmdes_lim = -1;
    error_flag_lim = MAX_SPROCKET;
end

% Limit motor movement in case of breakaway
if abs(pos_m) > 10*pi
    velmdes_lim = -1;
    error_flag_lim = MAX_MOTOR;
end

return

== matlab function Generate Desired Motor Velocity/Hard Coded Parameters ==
function p = params()

Rg = 5; % motor gear ratio
RgRf = 5*3.66/0.444; % total transmission gear ratio

Ks = 5.5*180/pi*0.113; % N m / rad, relationship between ankle torque and sprocket angle, all else constant
%%%%%^update Ks to below
%Ks = 14.89*180/pi*0.113; % N m / rad, relationship between ankle torque and sprocket angle, all else constant

Ka = -115.59*180/pi*0.113; % N m / rad, relationship between ankle torque and ankle angle, all else constant
%%%%%^update Ka to below
%Ka = -122.7278*180/pi*0.113; % N m / rad, relationship between ankle torque and ankle angle, all else constant

Ktr = inf;              % maybe 1000 N m / rad, stiffness between motor pulley and sprocket

p = [Rg RgRf Ks Ka Ktr];
